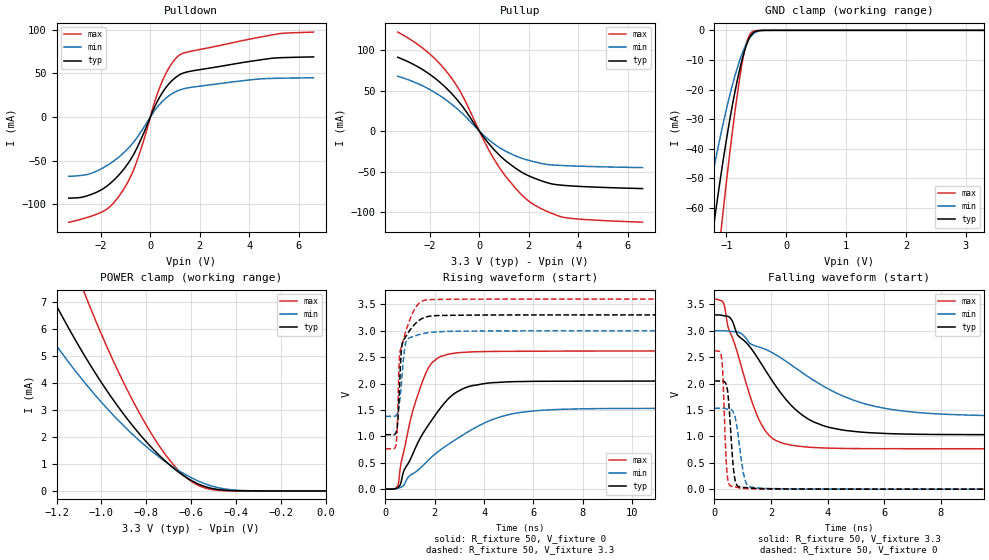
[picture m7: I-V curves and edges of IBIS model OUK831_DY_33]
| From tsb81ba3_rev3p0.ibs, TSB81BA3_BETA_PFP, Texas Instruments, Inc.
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[Model]   OUK831_DY_33
Model_type  3-state
Enable   Active-Low
Vref =   0
Rref =   500
Cref =   10p
Vmeas =   1.65
| variable   typ   min   max
C_comp   1.84pF   1.24pF   3.65pF
| C_pullup   4.20pF   1.90pF   4.97pF
| C_pulldown   4.41pF   1.09pF   6.96pF
| C_tri-state   1.84pF   1.24pF   3.65pF
[Temperature Range]   40   125   -40
| Ambient temperature   25   110   -40
[Voltage range]   3.3   3   3.6
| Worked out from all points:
|   slope of the pulldown table from 0 to 0.495 V, typ, clamps not added: 17.5 ohm
|   slope of the pullup table from 0 to 0.495 V, typ, clamps not added: 25.4 ohm
|   GND clamp passes 1 mA (typ) near -0.56 V on its own axis
|   POWER clamp passes 1 mA (typ) near -0.70 V on its own axis
|   rising waveform, R_fixture 50, V_fixture 0: 20-80 % time 1.6ns typ, 2.73ns min, 904ps max; typ from 0 V to 2.05 V
|   falling waveform, R_fixture 50, V_fixture 3.3: 20-80 % time 1.94ns typ, 3.16ns min, 1.06ns max; typ from 3.3 V to 1.03 V
|   rising waveform, R_fixture 50, V_fixture 3.3: 20-80 % time 234ps typ, 198ps min, 362ps max; typ from 1.03 V to 3.3 V
|   falling waveform, R_fixture 50, V_fixture 0: 20-80 % time 164ps typ, 242ps min, 114ps max; typ from 2.05 V to 0 V
[GND Clamp]
| OUK831_DY_33
|   Voltage   I(typ)   I(min)   I(max)
-3.3V     -464.3mA   -359.1mA   -569.6mA
-1.375V   -91.22mA   -65mA      -125.5mA
-1.205V   -64.93mA   -46.22mA   -90.3mA
-1.08V    -47.33mA   -33.86mA   -65.9mA
-895mV    -24.75mA   -18.17mA   -33.44mA
-750mV    -10.86mA   -8.573mA   -12.55mA
-705mV    -7.487mA   -6.229mA   -7.576mA
-655mV    -4.412mA   -4.063mA   -3.556mA
-610mV    -2.369mA   -2.55mA    -1.433mA
-550mV    -796.2uA   -1.185mA   -302.5uA
-240mV    -152.8nA   -1.997uA   -2.208nA
3.3V      147.9pA    2.865uA    18.25pA
[POWER Clamp]
| OUK831_DY_33
|   Voltage   I(typ)   I(min)   I(max)
-3.3V     61.52mA    46.8mA     83.31mA
-1.365V   9.625mA    7.405mA    14.24mA
-1.34V    9.181mA    7.079mA    13.58mA
-1.225V   7.245mA    5.66mA     10.7mA
-1.085V   5.142mA    4.116mA    7.52mA
-1.065V   4.866mA    3.913mA    7.1mA
-945mV    3.341mA    2.784mA    4.772mA
-810mV    1.911mA    1.71mA     2.577mA
-705mV    1.028mA    1.025mA    1.234mA
-615mV    461.9uA    556.2uA    447.9uA
-415mV    10.14uA    37.33uA    2.524uA
-48.03fV  147.9pA    5.993nA    21.92pA
[Pulldown]
| OUK831_DY_33
|   Voltage   I(typ)   I(min)   I(max)
-3.3V     -92.88mA   -67.99mA   -120.4mA
-2.645V   -90.96mA   -66.29mA   -115.7mA
-1.86V    -81.18mA   -57.4mA    -107.2mA
-1.145V   -62.21mA   -42.71mA   -85.6mA
-580mV    -37.66mA   -25.17mA   -53.29mA
-245mV    -16.92mA   -11.04mA   -24.58mA
185mV     12.21mA    7.772mA    18.2mA
445mV     25.97mA    16.58mA    38.53mA
790mV     39.09mA    24.99mA    57.83mA
1.15V     47.67mA    30.41mA    70.23mA
5.09V     67.52mA    44.19mA    94.67mA
6.6V      68.71mA    44.86mA    97.06mA
[Pullup]
| OUK831_DY_33
|   Voltage   I(typ)   I(min)   I(max)
-3.3V     90.98mA    67.61mA    122mA
-2.16V    73.12mA    53.66mA    99.03mA
-1.68V    62.31mA    45.28mA    85.55mA
-1.255V   50.51mA    36.29mA    70.62mA
-685mV    30.48mA    21.59mA    43.9mA
200mV     -8.372mA   -5.816mA   -12.54mA
705mV     -26.45mA   -18.13mA   -39.97mA
1.395V    -44.22mA   -29.67mA   -67.97mA
1.995V    -55.12mA   -36.09mA   -86.21mA
2.815V    -64.24mA   -41.39mA   -99.95mA
3.415V    -66.91mA   -42.54mA   -106.4mA
6.6V      -70.87mA   -45.01mA   -112.3mA
[Ramp]
| OUK831_DY_33
| variable   typ   min   max
dV/dt_r   1.23/1.60E-09   0.92/2.74E-09   1.57/9.07E-10
dV/dt_f   1.36/1.96E-09   0.97/3.18E-09   1.70/1.06E-09
R_load = 50
[Rising Waveform]
| OUK831_DY_33
R_fixture =   50
C_fixture =   0
L_fixture =   0
V_fixture =   0
V_fixture_min = 0
V_fixture_max = 0
|   Time   V(typ)   V(min)   V(max)
0s        -12.39uV   -75.96uV   -347.4nV
510ps     33.42mV    16.65mV    80mV
635ps     137.3mV    36.89mV    507.1mV
1.045ns   600.4mV    276.4mV    1.374V
1.69ns    1.18V      526.7mV    2.251V
2.11ns    1.462V     702.3mV    2.48V
2.66ns    1.76V      883.5mV    2.566V
4.665ns   2.024V     1.37V      2.609V
7.095ns   2.044V     1.512V     2.614V
40ns      2.049V     1.532V     2.619V
[Falling Waveform]
| OUK831_DY_33
R_fixture =   50
C_fixture =   0
L_fixture =   0
V_fixture =   3.3
V_fixture_min = 3
V_fixture_max = 3.6
|   Time   V(typ)   V(min)   V(max)
0s        3.3V       3V         3.6V
330ps     3.285V     3V         3.511V
495ps     3.268V     2.991V     3.046V
1.66ns    2.372V     2.678V     1.227V
2.115ns   1.995V     2.563V     937.8mV
2.875ns   1.504V     2.292V     820.2mV
3.85ns    1.202V     1.951V     780.4mV
5.2ns     1.08V      1.635V     768.1mV
8.2ns     1.035V     1.417V     765.7mV
40ns      1.032V     1.378V     765.2mV
[Rising Waveform]
| OUK831_DY_33
R_fixture =   50
C_fixture =   0
L_fixture =   0
V_fixture =   3.3
V_fixture_min = 3
V_fixture_max = 3.6
|   Time   V(typ)   V(min)   V(max)
0s        1.032V     1.377V     765.2mV
435ps     1.08V      1.4V       857mV
480ps     1.191V     1.437V     1.197V
550ps     1.705V     1.583V     2.361V
605ps     2.325V     1.795V     2.639V
680ps     2.749V     2.195V     2.749V
830ps     2.894V     2.783V     3.001V
1.225ns   3.142V     2.907V     3.441V
1.63ns    3.259V     2.955V     3.582V
40ns      3.3V       3V         3.6V
[Falling Waveform]
| OUK831_DY_33
R_fixture =   50
C_fixture =   0
L_fixture =   0
V_fixture =   0
V_fixture_min = 0
V_fixture_max = 0
|   Time   V(typ)   V(min)   V(max)
0s        2.049V     1.532V     2.619V
190ps     2.046V     1.533V     2.603V
270ps     2.043V     1.533V     2.401V
415ps     1.981V     1.521V     544.4mV
485ps     1.763V     1.514V     145.2mV
700ps     269.3mV    1.419V     51.36mV
950ps     36.79mV    549mV      17.49mV
1.19ns    25.86mV    59.77mV    9.061mV
1.94ns    6.791mV    12.79mV    2.929mV
40ns      2.479uV    2.882uV    1.968uV
